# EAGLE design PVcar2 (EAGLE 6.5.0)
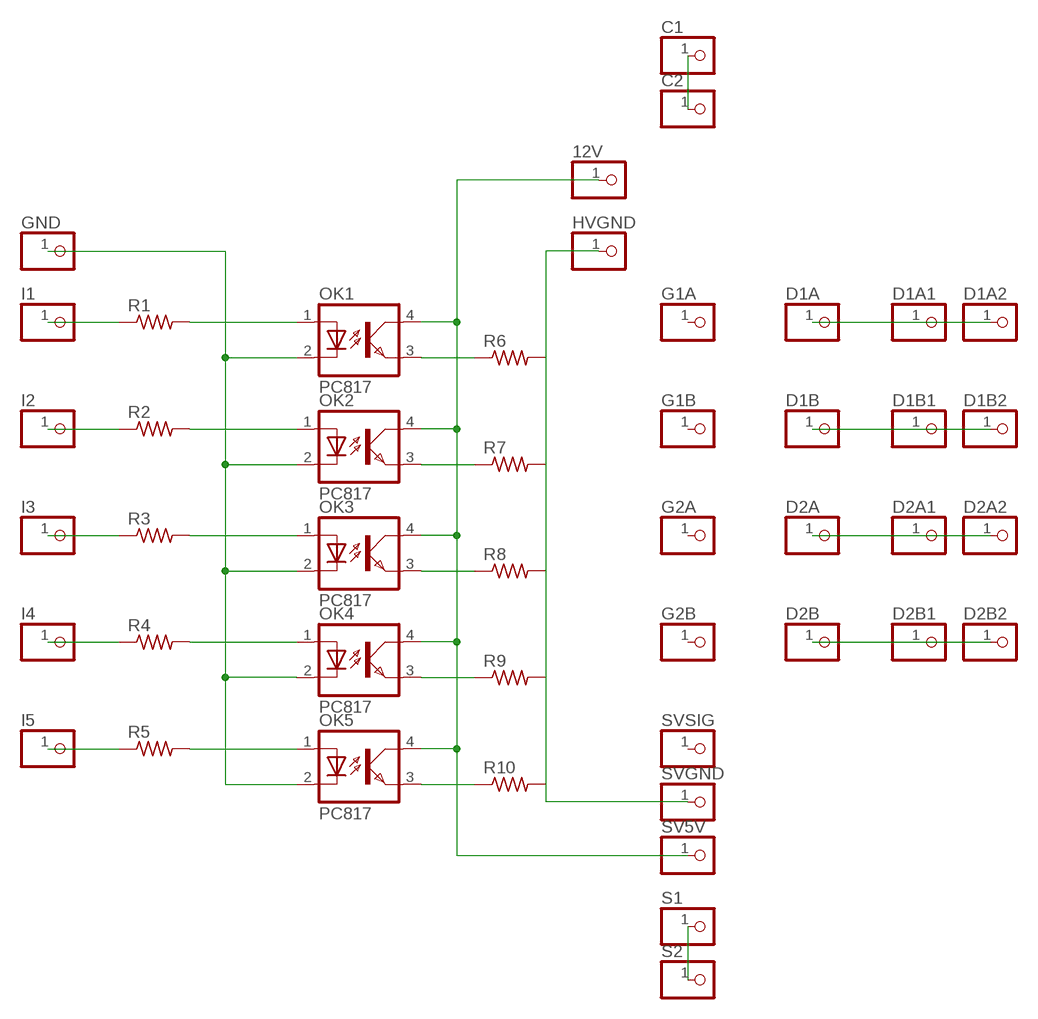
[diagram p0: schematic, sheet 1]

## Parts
12V  PINHD-1X1  [1X01]
C1  PINHD-1X1  [1X01]
C2  PINHD-1X1  [1X01]
D1A  PINHD-1X1  [1X01]
D1A1  PINHD-1X1  [1X01]
D1A2  PINHD-1X1  [1X01]
D1B  PINHD-1X1  [1X01]
D1B1  PINHD-1X1  [1X01]
D1B2  PINHD-1X1  [1X01]
D2A  PINHD-1X1  [1X01]
D2A1  PINHD-1X1  [1X01]
D2A2  PINHD-1X1  [1X01]
D2B  PINHD-1X1  [1X01]
D2B1  PINHD-1X1  [1X01]
D2B2  PINHD-1X1  [1X01]
G1A  PINHD-1X1  [1X01]
G1B  PINHD-1X1  [1X01]
G2A  PINHD-1X1  [1X01]
G2B  PINHD-1X1  [1X01]
GND  PINHD-1X1  [1X01]
HVGND  PINHD-1X1  [1X01]
I1  PINHD-1X1  [1X01]
I2  PINHD-1X1  [1X01]
I3  PINHD-1X1  [1X01]
I4  PINHD-1X1  [1X01]
I5  PINHD-1X1  [1X01]
OK1  PC817  [DIL04]
OK2  PC817  [DIL04]
OK3  PC817  [DIL04]
OK4  PC817  [DIL04]
OK5  PC817  [DIL04]
R1  R-US_0204/2V  [0204V]
R2  R-US_0204/2V  [0204V]
R3  R-US_0204/2V  [0204V]
R4  R-US_0204/2V  [0204V]
R5  R-US_0204/2V  [0204V]
R6  R-US_0204/2V  [0204V]
R7  R-US_0204/2V  [0204V]
R8  R-US_0204/2V  [0204V]
R9  R-US_0204/2V  [0204V]
R10  R-US_0204/2V  [0204V]
S1  PINHD-1X1  [1X01]
S2  PINHD-1X1  [1X01]
SV5V  PINHD-1X1  [1X01]
SVGND  PINHD-1X1  [1X01]
SVSIG  PINHD-1X1  [1X01]

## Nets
N$1: I1.1 R1.1
N$2: D1A1.1 D1A2.1 D1A.1
N$3: I2.1 R2.1
N$4: I3.1 R3.1
N$5: D1B1.1 D1B2.1 D1B.1
N$6: I4.1 R4.1
N$7: I5.1 R5.1
N$8: GND.1 OK1.2(C) OK2.2(C) OK3.2(C) OK4.2(C) OK5.2(C)
N$9: OK1.1(A) R1.2
N$10: OK2.1(A) R2.2
N$11: OK3.1(A) R3.2
N$12: OK4.1(A) R4.2
N$13: OK5.1(A) R5.2
N$14: OK1.3(EMIT) R6.1
N$15: OK2.3(EMIT) R7.1
N$16: OK3.3(EMIT) R8.1
N$17: OK4.3(EMIT) R9.1
N$18: 12V.1 OK1.4(COL) OK2.4(COL) OK3.4(COL) OK4.4(COL) OK5.4(COL) SV5V.1
N$19: HVGND.1 R6.2 R7.2 R8.2 R9.2 R10.2 SVGND.1
N$20: D2A1.1 D2A2.1 D2A.1
N$21: OK5.3(EMIT) R10.1
N$22: D2B1.1 D2B2.1 D2B.1
N$32: S1.1 S2.1
N$33: C1.1 C2.1
Unconnected: G1A.1 G1B.1 G2A.1 G2B.1 SVSIG.1

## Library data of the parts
12V C1 C2 D1A D1A1 D1A2 D1B D1B1 D1B2 D2A D2A1 D2A2 D2B D2B1 D2B2 G1A G1B G2A G2B GND HVGND I1-I5 S1 S2 SV5V SVGND SVSIG = pinhead:PINHD-1X1: PIN HEADER
OK1-OK5 = optocoupler:PC817: SHARP OPTO COUPLER; MPN: PC817X4J000F; OC_FARNELL: 9707727; OC_NEWARK: 97K7059
R1-R10 = resistor:R-US_: RESISTOR, American symbol

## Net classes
0 default: width 0.406 mm

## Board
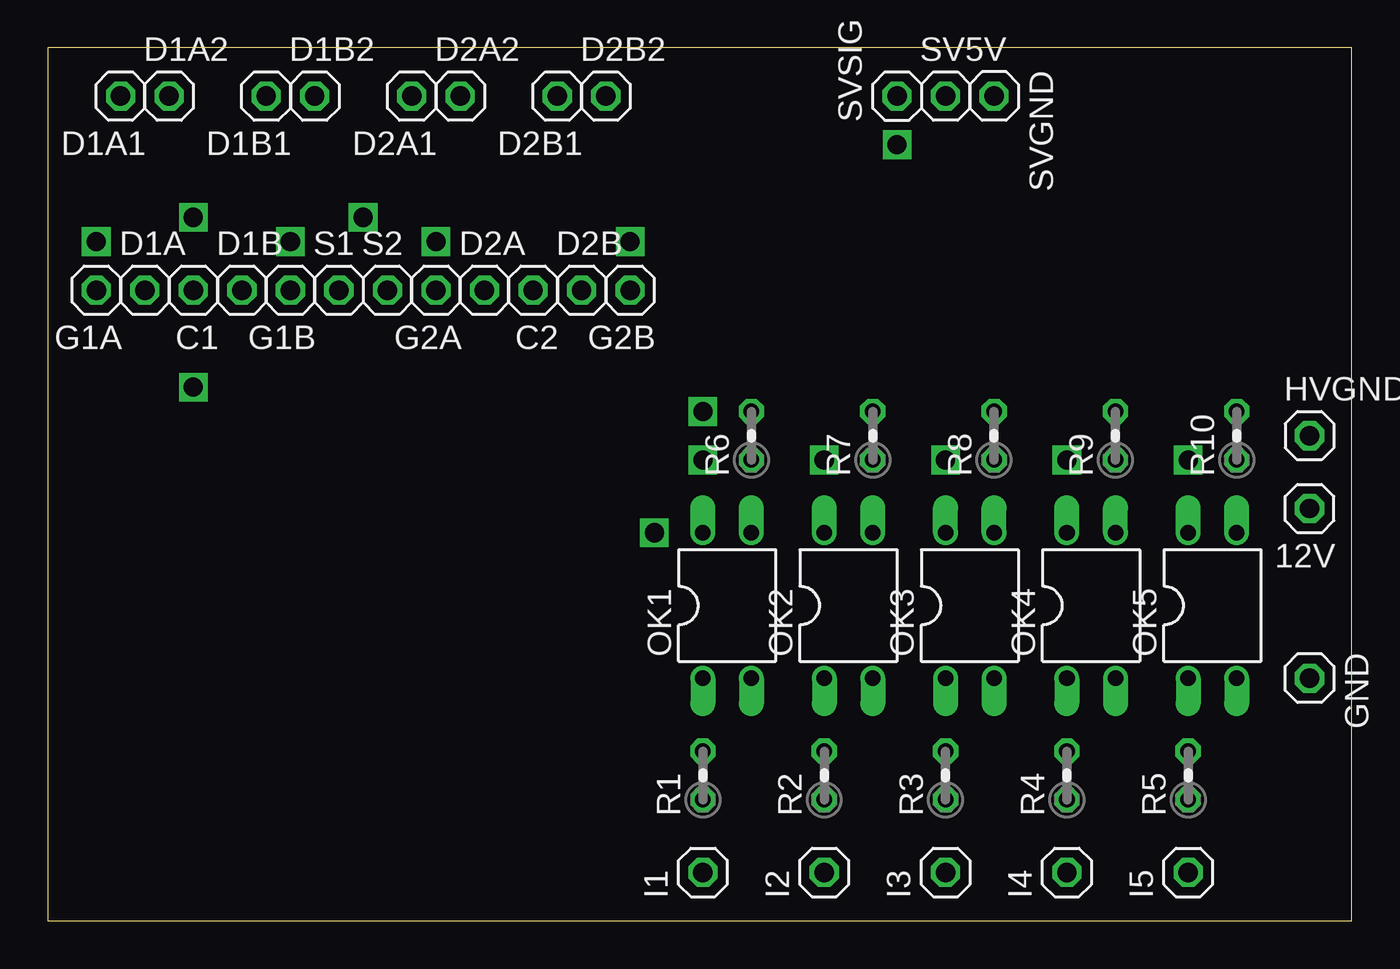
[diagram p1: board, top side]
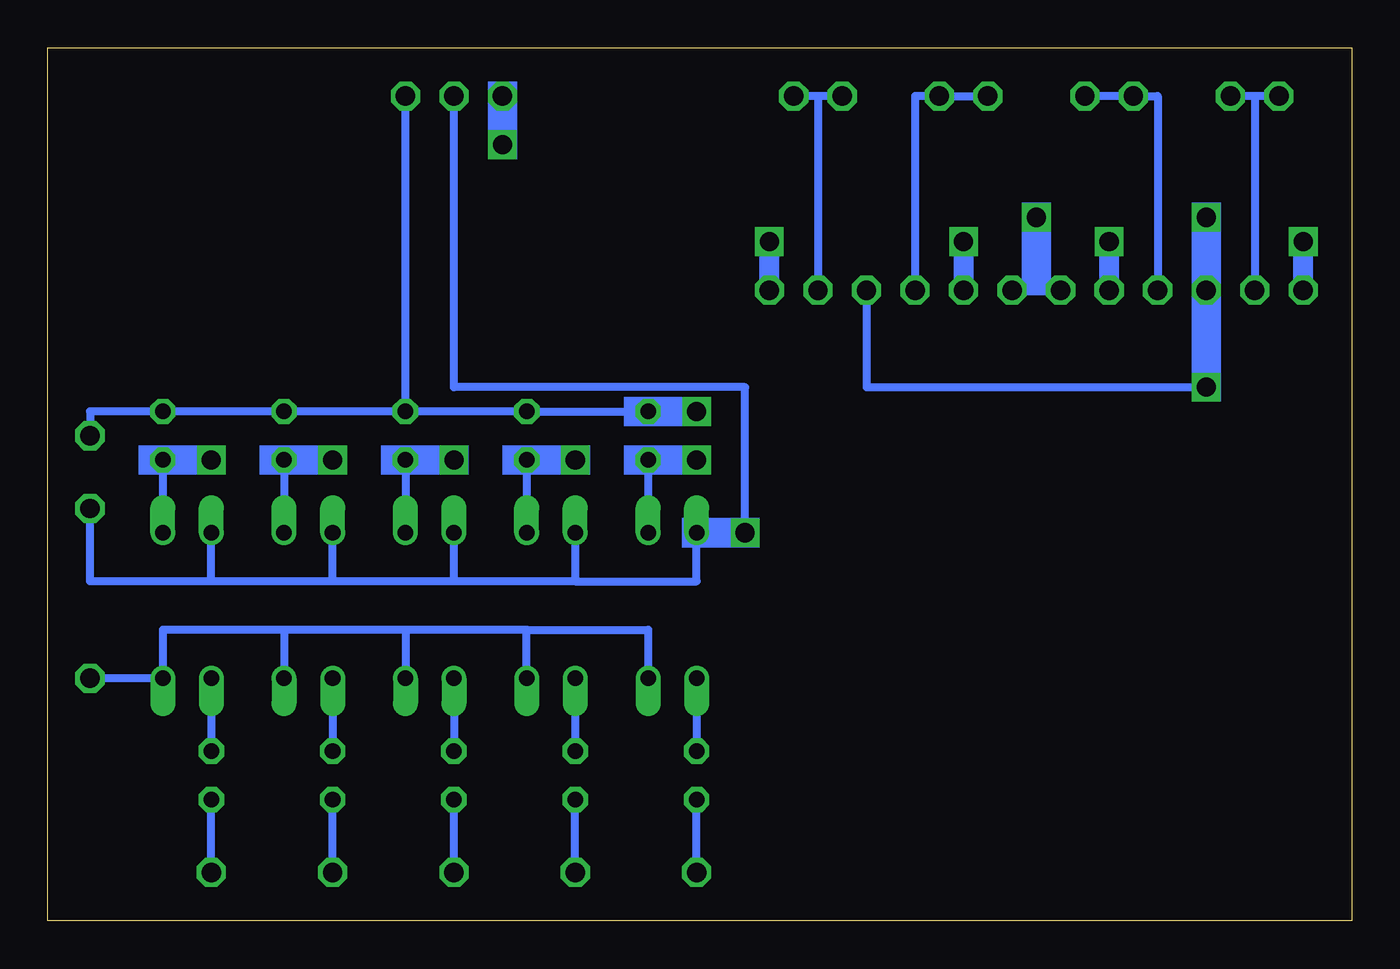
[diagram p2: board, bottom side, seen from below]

Size 68.25 x 45.71 mm. Coordinates in mm from the lower left corner, seen from the top.
Outline: 0,0 68.25,0 68.25,45.71 0,45.71 0,0
Copper layers (1*16): Top 0.035mm / dielectric 1.5mm / Bottom 0.035mm
Design rules "default": minimum track width 10mil, minimum drill 24mil, track to track 8mil, track to pad 8mil, pad to pad 8mil, via to via 8mil, smd to smd 8mil, copper to edge 40mil, drill to drill 8mil, minimum pad ring 10mil, minimum via ring 8mil, stop-mask expansion 4mil, vias tented up to drill 0mil, thermal gap 10mil

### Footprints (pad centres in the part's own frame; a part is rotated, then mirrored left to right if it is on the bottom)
1X01 = drill 1.016 octagon: 1 0,0
DIL04 = drill 0.813 offset: 1 -1.27,-3.81; 2 1.27,-3.81; 3 1.27,3.81; 4 -1.27,3.81
0204V = drill 0.813 octagon: 1 -1.27,0; 2 1.27,0

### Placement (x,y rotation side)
12V  66.04,21.59 180 top
C1  7.62,33.02 180 top
C2  25.4,33.02 180 top
D1A  5.08,33.02 0 top
D1A1  3.81,43.18 180 top
D1A2  6.35,43.18 0 top
D1B  10.16,33.02 0 top
D1B1  11.43,43.18 180 top
D1B2  13.97,43.18 0 top
D2A  22.86,33.02 0 top
D2A1  19.05,43.18 180 top
D2A2  21.59,43.18 0 top
D2B  27.94,33.02 0 top
D2B1  26.67,43.18 180 top
D2B2  29.21,43.18 0 top
G1A  2.54,33.02 180 top
G1B  12.7,33.02 180 top
G2A  20.32,33.02 180 top
G2B  30.48,33.02 180 top
GND  66.04,12.7 270 top
HVGND  66.04,25.4 0 top
I1  34.29,2.54 90 top
I2  40.64,2.54 90 top
I3  46.99,2.54 90 top
I4  53.34,2.54 90 top
I5  59.69,2.54 90 top
OK1  35.56,16.51 0 top
OK2  41.91,16.51 0 top
OK3  48.26,16.51 0 top
OK4  54.61,16.51 0 top
OK5  60.96,16.51 0 top
R1  34.29,7.62 90 top
R2  40.64,7.62 90 top
R3  46.99,7.62 90 top
R4  53.34,7.62 90 top
R5  59.69,7.62 90 top
R6  36.83,25.4 90 top
R7  43.18,25.4 90 top
R8  49.53,25.4 90 top
R9  55.88,25.4 90 top
R10  62.23,25.4 90 top
S1  15.24,33.02 0 top
S2  17.78,33.02 0 top
SV5V  46.99,43.18 0 top
SVGND  49.53,43.18 270 top
SVSIG  44.45,43.18 90 top

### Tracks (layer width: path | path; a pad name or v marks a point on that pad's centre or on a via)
N$1
  Bottom 0.406: I1.1 R1.1
N$2
  Bottom 0.406: 5.08,43.18 D1A.1 | D1A1.1 5.08,43.18 | 5.08,43.18 D1A2.1
N$3
  Bottom 0.406: I2.1 R2.1
N$4
  Bottom 0.406: I3.1 R3.1
N$5
  Bottom 0.406: D1B.1 10.16,43.18 D1B1.1 D1B2.1
N$6
  Bottom 0.406: I4.1 R4.1
N$7
  Bottom 0.406: I5.1 R5.1
N$8
  Bottom 0.406: OK1.2 36.83,15.24 43.18,15.24 | OK2.2 43.18,15.24 | 49.53,15.24 OK3.2 | 43.18,15.24 49.53,15.24 | 55.88,15.24 OK4.2 | 49.53,15.24 55.88,15.24 | 55.88,15.24 62.23,15.24 OK5.2 GND.1
N$9
  Bottom 0.406: OK1.1 R1.2
N$10
  Bottom 0.406: OK2.1 R2.2
N$11
  Bottom 0.406: OK3.1 R3.2
N$12
  Bottom 0.406: OK4.1 R4.2
N$13
  Bottom 0.406: OK5.1 R5.2
N$14
  Bottom 0.406: R6.1 OK1.3
N$15
  Bottom 0.406: R7.1 OK2.3
N$16
  Bottom 0.406: R8.1 OK3.3
N$17
  Bottom 0.406: R9.1 OK4.3
N$18  (via drill 1)
  Bottom 0.406: 40.64,17.78 34.29,17.78 OK1.4 v31.75,20.32 31.75,27.94 46.99,27.94 SV5V.1 | OK2.4 40.64,17.78 | 46.99,17.78 OK3.4 | 40.64,17.78 46.99,17.78 | 53.34,17.78 OK4.4 | 46.99,17.78 53.34,17.78 | 59.69,17.78 OK5.4 | 53.34,17.78 59.69,17.78 | 12V.1 66.04,17.78 59.69,17.78
N$19
  Bottom 0.406: R6.2 R7.2 R8.2 | R8.2 R9.2 R10.2 66.04,26.67 HVGND.1 | R8.2 SVGND.1
N$20
  Bottom 0.406: D2A.1 22.86,43.18 D2A2.1 D2A1.1
N$21
  Bottom 0.406: R10.1 OK5.3
N$22
  Bottom 0.406: 27.94,43.18 D2B.1 | D2B1.1 27.94,43.18 | 27.94,43.18 D2B2.1
N$23  (via drill 1)
  other vias: 2.54,35.56
N$24  (via drill 1)
  other vias: 12.7,35.56
N$25  (via drill 1)
  other vias: 20.32,35.56
N$26  (via drill 1)
  other vias: 30.48,35.56
N$27  (via drill 1)
  other vias: 34.29,24.13
N$28  (via drill 1)
  other vias: 40.64,24.13
N$29  (via drill 1)
  other vias: 46.99,24.13
N$30  (via drill 1)
  other vias: 53.34,24.13
N$31  (via drill 1)
  other vias: 59.69,24.13
N$32
  Bottom 0.406: S2.1 S1.1
N$33  (via drill 1)
  Bottom 0.406: C1.1 v7.62,27.94 25.4,27.94 C2.1
N$34  (via drill 1)
  other vias: 44.45,40.64
N$35  (via drill 1)
  other vias: 34.29,26.67
N$36  (via drill 1)
  other vias: 16.51,36.83
N$37  (via drill 1)
  other vias: 7.62,36.83
(copper drawn outside any net)
  shapes: Bottom area x14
